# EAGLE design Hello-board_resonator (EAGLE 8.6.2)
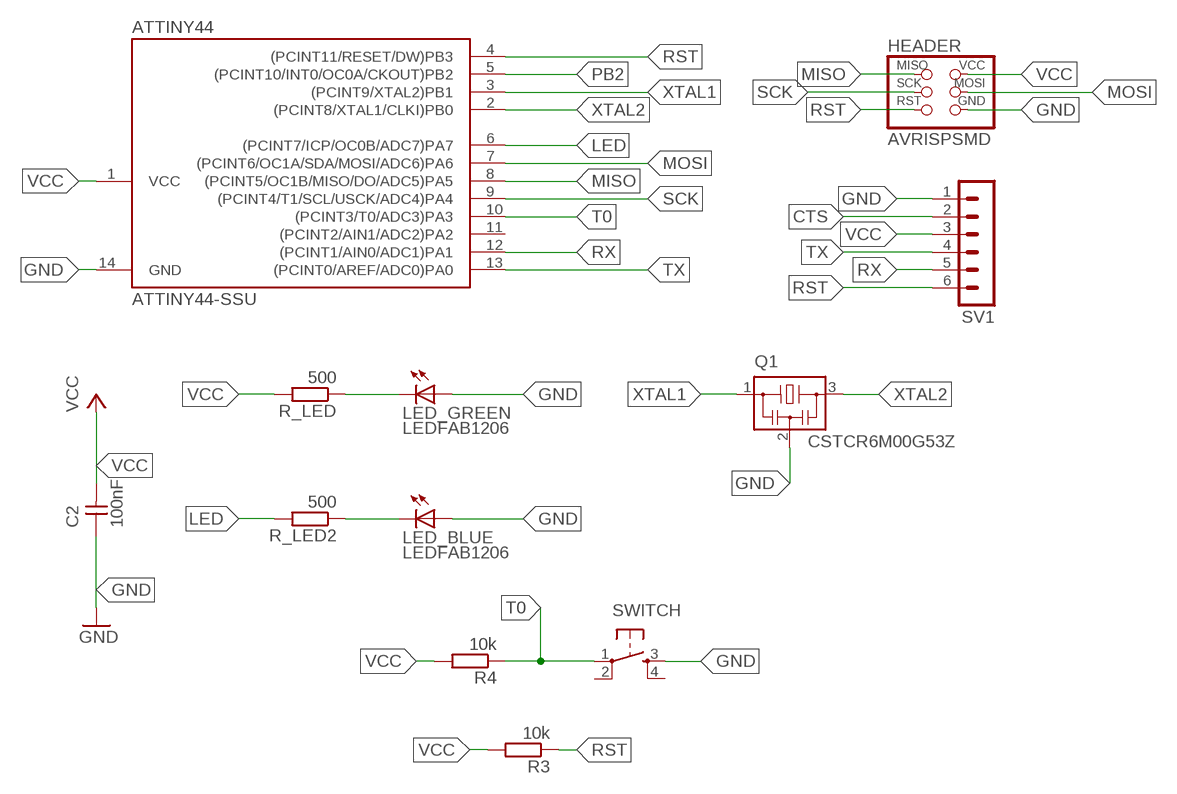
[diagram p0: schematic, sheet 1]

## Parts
ATTINY44  ATTINY44-SSU  [SOIC14]
C2  100nF  CAP-UNPOLARIZEDFAB  [C1206FAB]
HEADER  AVRISPSMD  [2X03SMD]
LED_BLUE  LEDFAB1206  [LED1206FAB]
LED_GREEN  LEDFAB1206  [LED1206FAB]
Q1  CSTCR6M00G53Z  [CSTCR6M]
R3  10k  R-EU_R1206  [R1206]
R4  10k  R-EU_R1206  [R1206]
R_LED  500  R-EU_R1206  [R1206]
R_LED2  500  R-EU_R1206  [R1206]
SV1  MA06-1  [MA06-1]
SWITCH  6MM_SWITCH6MM_SWITCH  [6MM_SWITCH]

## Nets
CTS: SV1.2
GND: ATTINY44.14(GND) C2.1 HEADER.6(GND) LED_BLUE.1(A) LED_GREEN.1(A) Q1.2 SV1.1 SWITCH.3(S)
LED: ATTINY44.6((PCINT7/ICP/OC0B/ADC7)PA7) R_LED2.2
MISO: ATTINY44.8((PCINT5/OC1B/MISO/DO/ADC5)PA5) HEADER.1(MISO)
MOSI: ATTINY44.7((PCINT6/OC1A/SDA/MOSI/ADC6)PA6) HEADER.4(MOSI)
N$21: LED_GREEN.2(C) R_LED.1
N$22: LED_BLUE.2(C) R_LED2.1
PB2: ATTINY44.5((PCINT10/INT0/OC0A/CKOUT)PB2)
RST: ATTINY44.4((PCINT11/RESET/DW)PB3) HEADER.5(RST) R3.1 SV1.6
RX: ATTINY44.12((PCINT1/AIN0/ADC1)PA1) SV1.5
SCK: ATTINY44.9((PCINT4/T1/SCL/USCK/ADC4)PA4) HEADER.3(SCK)
T0: ATTINY44.10((PCINT3/T0/ADC3)PA3) R4.1 SWITCH.1(P)
TX: ATTINY44.13((PCINT0/AREF/ADC0)PA0) SV1.4
VCC: ATTINY44.1(VCC) C2.2 HEADER.2(VCC) R3.2 R4.2 R_LED.2 SV1.3
XTAL1: ATTINY44.3((PCINT9/XTAL2)PB1) Q1.1
XTAL2: ATTINY44.2((PCINT8/XTAL1/CLKI)PB0) Q1.3
Unconnected: ATTINY44.11((PCINT2/AIN1/ADC2)PA2) SWITCH.2(P1) SWITCH.4(S1)

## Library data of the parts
ATTINY44 = fab:ATTINY44
C2 = fab:CAP-UNPOLARIZED
HEADER = fab:AVRISP
LED_BLUE LED_GREEN = fab:LED: LED
Q1 = murata-filter:CSTCR: Resonator Source: murata.co.jp; MPN: CSTCR6M00G53-R0; OC_FARNELL: 1170434; OC_NEWARK: 25M8759
R3 R4 R_LED R_LED2 = resistor:R-EU_: RESISTOR, European symbol
SV1 = con-lstb:MA06-1: PIN HEADER; OC_FARNELL: unknown; OC_NEWARK: unknown
SWITCH = fab:6MM_SWITCH: OMRON SWITCH

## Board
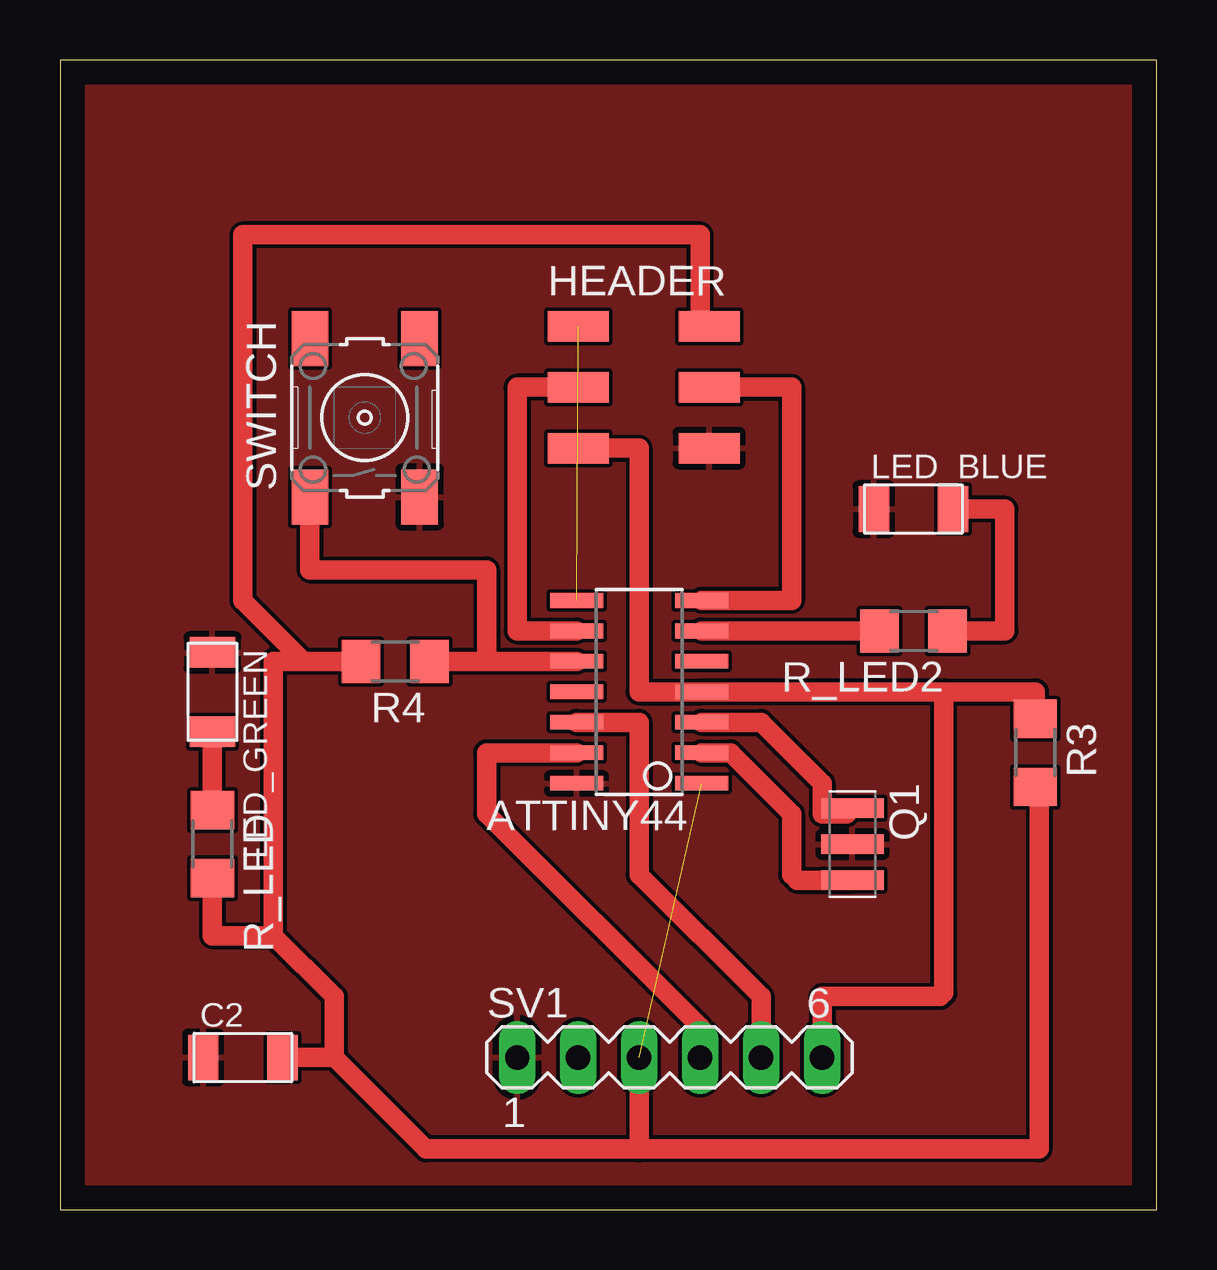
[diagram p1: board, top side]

Size 45.7 x 47.93 mm. Coordinates in mm from the lower left corner, seen from the top.
Outline: 0,0 45.7,0 45.7,47.93 0,47.93 0,0
Copper layers (1*16): Top 0.035mm / dielectric 1.5mm / Bottom 0.035mm
Design rules "default": minimum track width 6mil, minimum drill 0.35mm, track to track 6mil, track to pad 6mil, pad to pad 6mil, via to via 6mil, smd to smd 6mil, copper to edge 40mil, drill to drill 6mil, minimum pad ring 10mil, minimum via ring 8mil, stop-mask expansion 4mil, vias tented up to drill 0mil, thermal gap 10mil

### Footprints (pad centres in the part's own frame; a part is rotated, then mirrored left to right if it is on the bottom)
SOIC14 = smd 0.61 x 2.21: 1 -3.81,-2.603; 2 -2.54,-2.603; 3 -1.27,-2.603; 4 0,-2.603; 5 1.27,-2.603; 6 2.54,-2.603; 7 3.81,-2.603; 8 3.81,2.603; 9 2.54,2.603; 10 1.27,2.603; 11 0,2.603; 12 -1.27,2.603; 13 -2.54,2.603; 14 -3.81,2.603
C1206FAB = smd 1.27 x 1.905: 1 -1.651,0; 2 1.651,0
2X03SMD = smd 2.54 x 1.27: 1 -2.54,2.54; 2 2.92,2.54; 3 -2.54,0; 4 2.92,0; 5 -2.54,-2.54; 6 2.92,-2.54
LED1206FAB = smd 1.27 x 1.905: 1 -1.651,0; 2 1.651,0
CSTCR6M = smd 0.8 x 2.6: 1 -1.5,0; 2 0,0; 3 1.5,0
R1206 = smd 1.6 x 1.803: 1 -1.422,0; 2 1.422,0
MA06-1 = drill 1.016 long: 1 -6.35,0; 2 -3.81,0; 3 -1.27,0; 4 1.27,0; 5 3.81,0; 6 6.35,0
6MM_SWITCH = smd 2.286 x 1.524: 1 -3.302,2.286; 2 3.302,2.286; 3 -3.302,-2.286; 4 3.302,-2.286

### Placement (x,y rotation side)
ATTINY44  24.13,21.59 90 top
C2  7.62,6.35 0 top
HEADER  24.13,34.29 0 top
LED_BLUE  35.56,29.21 0 top
LED_GREEN  6.35,21.59 270 top
Q1  33.02,15.24 270 top
R3  40.64,19.05 270 top
R4  13.97,22.86 180 top
R_LED  6.35,15.24 270 top
R_LED2  35.56,24.13 180 top
SV1  25.4,6.35 0 top
SWITCH  12.7,33.02 90 top

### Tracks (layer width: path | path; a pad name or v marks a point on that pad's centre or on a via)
GND
  pour Top: -1.27,52.07 -1.27,-3.81 53.34,-3.81 53.34,52.07
LED
  Top 0.813: ATTINY44.6 R_LED2.2
MISO  (1 unrouted)
MOSI
  Top 0.813: HEADER.4 30.48,34.29 30.48,25.4 ATTINY44.7
N$21
  Top 0.813: R_LED.1 LED_GREEN.2
N$22
  Top 0.813: R_LED2.1 39.37,24.13 39.37,29.21 LED_BLUE.2
RST
  Top 0.813: SV1.6 31.75,8.89 36.68,8.89 36.83,9.04 36.83,21.59 | HEADER.5 24.13,31.75 24.13,21.59 ATTINY44.4 36.83,21.59 | 36.83,21.59 40.64,21.59 R3.1
RX
  Top 0.813: ATTINY44.12 24.13,20.32 24.13,13.97 29.21,8.89 SV1.5
SCK
  Top 0.813: HEADER.3 19.05,34.29 19.05,24.13 ATTINY44.9
T0
  Top 0.813: ATTINY44.10 17.78,22.86 | 17.78,22.86 R4.1 | SWITCH.1 10.41,26.67 17.78,26.67 17.78,22.86
TX
  Top 0.813: ATTINY44.13 17.78,19.05 17.78,16.51 26.67,7.62 SV1.4
VCC  (1 unrouted)
  Top 0.813: SV1.3 24.13,2.54 | 24.13,2.54 15.24,2.54 11.43,6.35 | 11.43,6.35 C2.2 | R_LED.2 6.35,11.43 8.89,11.43 | 8.89,11.43 11.43,8.89 11.43,6.35 | R4.2 10.16,22.86 | 10.16,22.86 8.89,22.86 8.89,11.43 | 24.13,2.54 40.79,2.54 40.79,17.48 R3.2 | HEADER.2 26.67,37.21 26.67,40.64 7.62,40.64 7.62,25.4 10.16,22.86
XTAL1
  Top 0.813: ATTINY44.3 29.21,20.32 31.75,17.78 31.75,16.51 32.79,16.51 Q1.1
XTAL2
  Top 0.813: ATTINY44.2 27.94,19.05 30.48,16.51 30.48,13.97 30.71,13.74 Q1.3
